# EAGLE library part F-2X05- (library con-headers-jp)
FEMALE HEADER
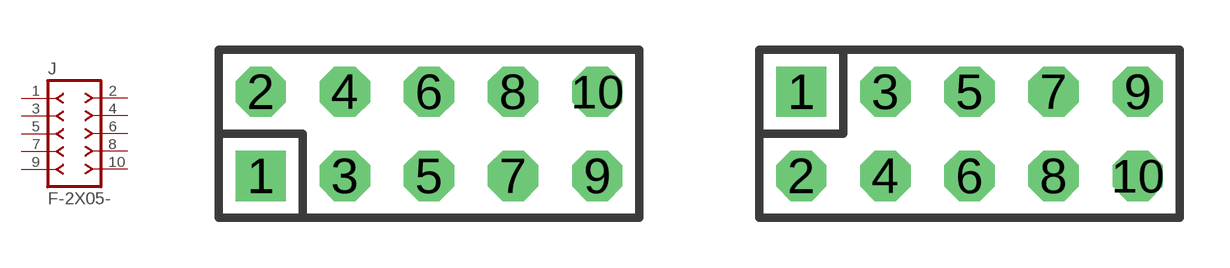
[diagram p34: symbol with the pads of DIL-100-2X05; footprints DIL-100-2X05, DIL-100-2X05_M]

Designator prefix J

## F-2X05-DIL-100  [DIL-100-2X05]
1  1  pas
2  2  pas
3  3  pas
4  4  pas
5  5  pas
6  6  pas
7  7  pas
8  8  pas
9  9  pas
10  10  pas

## F-2X05-DIL-100_M  [DIL-100-2X05_M]
Pads as for DIL-100-2X05

## F-2X05-DIL-2MM  [DIL-2MM-2X05]
Pads as for DIL-100-2X05

## F-2X05-DIL-2MM_M  [DIL-2MM-2X05_M]
Pads as for DIL-100-2X05

## F-2X05-71991  [71991-10]
Pads as for DIL-100-2X05

## F-2X05-79107  [79107-10]
Pads as for DIL-100-2X05

## F-2X05-79107_M  [79107-10_M]
Pads as for DIL-100-2X05

## Footprint DIL-100-2X05 (pad centres in mm)
PIN HEADER - 0.1"
drill 1.016 square: 1 -5.08,-1.27
drill 1.016 octagon: 2 -5.08,1.27; 3 -2.54,-1.27; 4 -2.54,1.27; 5 0,-1.27; 6 0,1.27; 7 2.54,-1.27; 8 2.54,1.27; 9 5.08,-1.27; 10 5.08,1.27

## Footprint DIL-100-2X05_M (pad centres in mm)
PIN HEADER - MIRRORED 0.1"
drill 1.016 square: 1 -5.08,1.27
drill 1.016 octagon: 2 -5.08,-1.27; 3 -2.54,1.27; 4 -2.54,-1.27; 5 0,1.27; 6 0,-1.27; 7 2.54,1.27; 8 2.54,-1.27; 9 5.08,1.27; 10 5.08,-1.27

## Footprint DIL-2MM-2X05 (pad centres in mm)
PIN HEADER - 2MM"
drill 0.711 square: 1 -4,-1
drill 0.711: 2 -4,1; 3 -2,-1; 4 -2,1; 5 0,-1; 6 0,1; 7 2,-1; 8 2,1; 9 4,-1; 10 4,1

## Footprint DIL-2MM-2X05_M (pad centres in mm)
PIN HEADER - MIRRORED 2MM
drill 0.711 square: 1 -4,1
drill 0.711: 2 -4,-1; 3 -2,1; 4 -2,-1; 5 0,1; 6 0,-1; 7 2,1; 8 2,-1; 9 4,1; 10 4,-1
